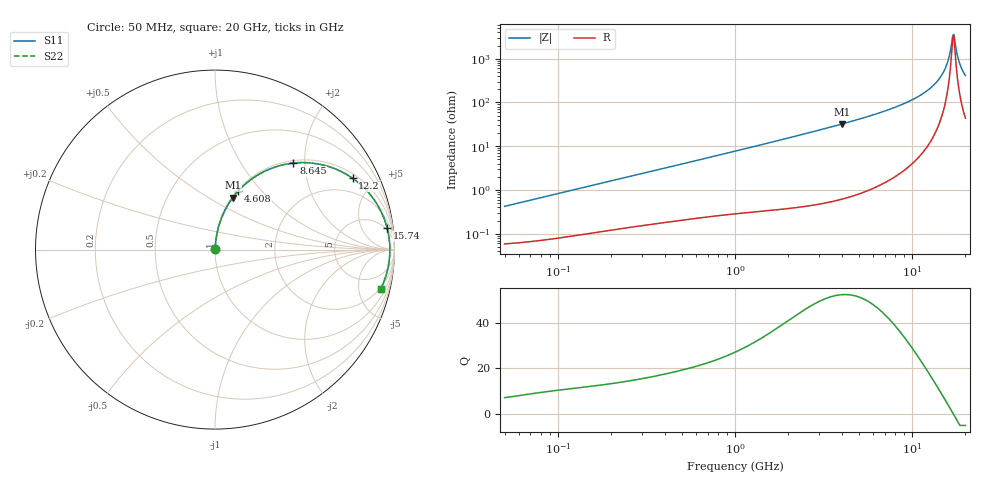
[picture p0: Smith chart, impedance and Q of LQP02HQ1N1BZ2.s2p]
!Murata Part Number: LQP02HQ1N1BZ2
!These Parameters are Measured in Series Mode Connection
!  o--[Z]--o
!Port1  Port2
!  o-------o
!Freq. Start=50[MHz] Stop=20[GHz], 401[Steps]
# Hz S RI R 50
!Freq.(Hz) S11(Real) S11(Imag) S21(Real) S21(Imag) S12(Real) S12(Imag) S22(Real) S22(Imag)
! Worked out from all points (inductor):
!   401 points, 50 MHz to 20 GHz, reference 50 ohm
!   read as one part in series: L = 1.33 nH near 51.52 MHz
!   highest Q = 52.3 at 4.027 GHz (marker M1), where L = 1.28 nH
!   self-resonance near 16.96 GHz
!   S11 on the Smith chart (normalised r, x): 50 MHz: 1.00, +0.01; 4.608 GHz: 1.01, +0.75; 8.645 GHz: 1.05, +1.76; 12.2 GHz: 1.20, +3.75; 15.74 GHz: 4, +15; 20 GHz: 1.87, -8.18
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5e7  0.000602 0.00418  0.9994 -0.00418  0.9994 -0.00418  0.000602 0.00418
1.364002e8  0.00108 0.0111  0.9989 -0.0111  0.9989 -0.0111  0.00108 0.0111
3.721004e8  0.00258 0.0292  0.9974 -0.0292  0.9974 -0.0292  0.00258 0.0292
1e9  0.00868 0.0761  0.9913 -0.0761  0.9913 -0.0761  0.00868 0.0761
2.728004e9  0.047 0.2015  0.953 -0.2015  0.953 -0.2015  0.047 0.2015
4.026975e9  0.099 0.2892  0.901 -0.2892  0.901 -0.2892  0.099 0.2892
4.608136e9  0.1288 0.3255  0.8712 -0.3255  0.8712 -0.3255  0.1288 0.3255
7.442007e9  0.3294 0.4581  0.6706 -0.4581  0.6706 -0.4581  0.3294 0.4581
8.644534e9  0.4373 0.4822  0.5627 -0.4822  0.5627 -0.4822  0.4373 0.4822
1.034674e10  0.6 0.4719  0.4 -0.4719  0.4 -0.4719  0.6 0.4719
1.220001e10  0.7669 0.3972  0.2331 -0.3972  0.2331 -0.3972  0.7669 0.3972
1.417136e10  0.9003 0.2567  0.0997 -0.2567  0.0997 -0.2567  0.9003 0.2567
1.504638e10  0.9385 0.1821  0.0615 -0.1821  0.0615 -0.1821  0.9385 0.1821
1.573793e10  0.9588 0.1209  0.0412 -0.1209  0.0412 -0.1209  0.9588 0.1209
1.621653e10  0.9678 0.0784  0.0322 -0.0784  0.0322 -0.0784  0.9678 0.0784
1.670968e10  0.973 0.0349  0.027 -0.0349  0.027 -0.0349  0.973 0.0349
1.696185e10  0.9742 0.013  0.0258 -0.013  0.0258 -0.013  0.9742 0.013
1.721783e10  0.9743 -0.00895  0.0257 0.00895  0.0257 0.00895  0.9743 -0.00895
1.747767e10  0.9735 -0.0309  0.0265 0.0309  0.0265 0.0309  0.9735 -0.0309
1.855685e10  0.9604 -0.1172  0.0396 0.1172  0.0396 0.1172  0.9604 -0.1172
1.940974e10  0.9408 -0.1788  0.0592 0.1788  0.0592 0.1788  0.9408 -0.1788
2e10  0.9236 -0.2176  0.0764 0.2176  0.0764 0.2176  0.9236 -0.2176
